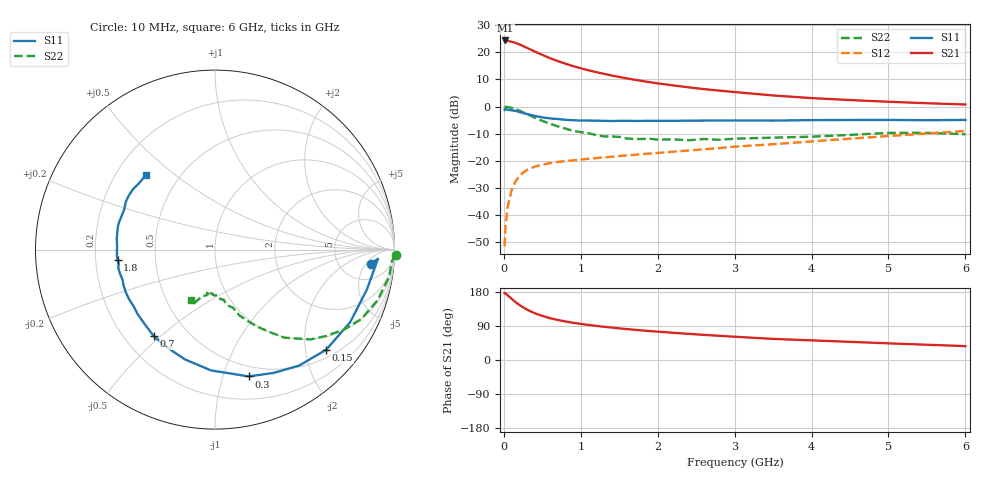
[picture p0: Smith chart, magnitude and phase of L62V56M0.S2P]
!  INFINEON TECHNOLOGIES Small Signal Semiconductors
! BFR380L3 , Si-NPN RF-Transistor in TSLP-3-1
!  Vce=2.5 V,  Ic=6 mA
! Common Emitter S-Parameters:  07. March 2005
#  GHz  S  MA  R  50
! f  S11  S21  S12  S22
! GHz  Mag  Ang  Mag  Ang  Mag  Ang  Mag  Ang
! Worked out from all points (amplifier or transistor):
!   36 points, 10 MHz to 6 GHz, reference 50 ohm
!   highest |S21| = 24.3 dB at 20 MHz (marker M1)
!   |S21| within 3 dB of that: start of sweep to 320.9 MHz
!   unconditionally stable (mu >= 1): 2.305 GHz to 4.743 GHz
!   at 250 MHz: K = 0.19, MSG = 23.3 dB, |S12| = -24.3 dB
!   at 1.4 GHz: K = 0.80, MSG = 15.0 dB, |S12| = -18.5 dB
!   at 6 GHz: K = 0.95, MSG = 4.9 dB, |S12| = -9.0 dB
!   S11 on the Smith chart (normalised r, x): 10 MHz: 10, -7; 150 MHz: 0.67, -2.45; 300 MHz: 0.40, -1.22; 700 MHz: 0.32, -0.47; 1.8 GHz: 0.30, -0.05; 6 GHz: 0.32, +0.40
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0.01  0.8702 -5.3  16.4 176.4  0.0027 79.2  1.01 -1.8
0.02  0.9095 -3.2  16.48 176.4  0.0059 91.1  0.9876 -3.6
0.05  0.8752 -14.7  16.2 170.6  0.0143 82.4  0.9821 -8.8
0.1  0.8549 -28.2  15.62 161.8  0.0289 76.5  0.9489 -17.3
0.15  0.8338 -42.0  14.93 153.2  0.0418 68.8  0.9023 -25.4
0.2  0.7982 -54.1  13.98 145.5  0.0519 63.9  0.8465 -31.7
0.25  0.7603 -64.7  13.01 139.1  0.0608 59.4  0.7827 -38.0
0.3  0.7312 -75.1  12.04 133.0  0.0682 55.3  0.7312 -43.2
0.4  0.6734 -91.9  10.36 123.5  0.0785 49.7  0.6256 -51.7
0.5  0.6343 -105.3  8.94 116.4  0.0853 46.5  0.5454 -56.9
0.6  0.6058 -116.7  7.776 110.3  0.0911 44.2  0.4842 -61.7
0.7  0.5909 -125.3  6.886 105.8  0.0959 43.5  0.4336 -65.7
0.9  0.5612 -140.3  5.553 98.2  0.1024 42.4  0.3577 -71.8
1.1  0.5528 -150.0  4.655 92.5  0.1099 43.3  0.3231 -76.2
1.4  0.5417 -161.9  3.731 85.7  0.1191 44.9  0.2829 -81.3
1.8  0.5452 -174.1  2.96 77.9  0.1333 48.2  0.2536 -88.1
2.2  0.5462 177.4  2.454 71.8  0.1479 51.0  0.2495 -92.8
2.8  0.5562 166.5  1.967 63.9  0.1721 55.1  0.2445 -100.5
3.5  0.5524 156.4  1.601 55.7  0.2032 57.1  0.2684 -104.7
4.5  0.5667 148.2  1.318 47.9  0.2567 60.2  0.3011 -109.3
5.5  0.5617 138.5  1.153 40.3  0.32 59.8  0.3287 -113.5
6  0.5675 132.5  1.093 36.6  0.3552 58.6  0.3095 -116.0
